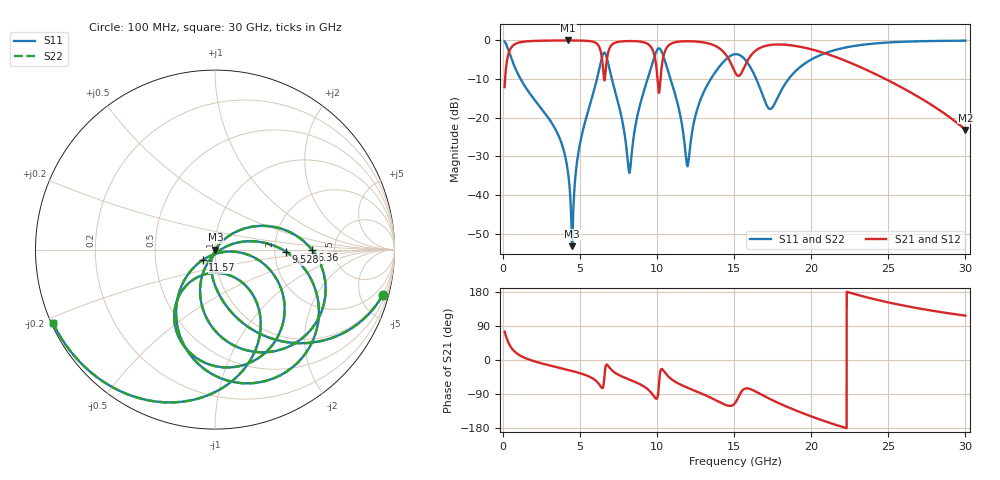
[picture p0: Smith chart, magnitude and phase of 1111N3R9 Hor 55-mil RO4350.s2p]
# GHz S MA R 50
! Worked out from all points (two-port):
!   3201 points, 100 MHz to 30 GHz, reference 50 ohm
!   highest |S21| = -0.02 dB at 4.221 GHz (marker M1); lowest = -23.2 dB at 30 GHz (marker M2)
!   |S21| within 3 dB of the highest: 388.2 MHz to 6.346 GHz (5.957 GHz wide, 177 % of centre); 16.28 GHz to 20.64 GHz (4.351 GHz wide, 23.6 % of centre)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
!   lowest |S11| = -53.3 dB at 4.482 GHz (marker M3), VSWR 1.00, Z = 50.2 - j0.11 ohm
!   |S11| at or under -10 dB: 1.14 GHz to 6.091 GHz (4.951 GHz wide, 137 % of centre); 7.061 GHz to 9.377 GHz (2.316 GHz wide, 28.2 % of centre); 10.87 GHz to 13.48 GHz (2.61 GHz wide, 21.4 % of centre)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
!   |S22| runs from -53.3 to -0.1 dB; largest |S21 - S12| = 0
!   S11 on the Smith chart (normalised r, x): 100 MHz: 0.92, -7.46; 6.36 GHz: 3.36, -0.02; 9.528 GHz: 2.31, -0.07; 11.57 GHz: 0.87, -0.10; 30 GHz: 0.00, -0.22
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0.1  0.9686 -15.0  0.2484 74.9  0.2484 74.9  0.9686 -15.0
1.081094  0.3325 -77.6  0.9424 12.3  0.9424 12.3  0.3325 -77.6
3.482438  0.0656 -107.9  0.9962 -18.9  0.9962 -18.9  0.0656 -107.9
4.220594  0.01912 -110.9  0.9975 -26.3  0.9975 -26.3  0.01912 -110.9
4.482219  0.002174 -30.4  0.9973 -29.0  0.9973 -29.0  0.002174 -30.4
5.089563  0.05712 49.7  0.9936 -36.1  0.9936 -36.1  0.05712 49.7
6.360313  0.5411 -0.2  0.6844 -71.5  0.6844 -71.5  0.5411 -0.2
6.724719  0.6008 -70.5  0.5441 -12.0  0.5441 -12.0  0.6008 -70.5
7.089125  0.3005 -105.0  0.8874 -28.0  0.8874 -28.0  0.3005 -105.0
8.191688  0.01933 -52.8  0.9798 -51.6  0.9798 -51.6  0.01933 -52.8
9.527844  0.3967 -1.8  0.8551 -82.5  0.8551 -82.5  0.3967 -1.8
10.06978  0.7833 -55.4  0.2419 -86.2  0.2419 -86.2  0.7833 -55.4
10.55566  0.5029 -113.6  0.7632 -35.8  0.7632 -35.8  0.5029 -113.6
11.57413  0.08905 -139.6  0.9698 -66.1  0.9698 -66.1  0.08905 -139.6
11.98525  0.02383 -63.4  0.9752 -73.5  0.9752 -73.5  0.02383 -63.4
12.98503  0.2067 -10.2  0.9426 -90.5  0.9426 -90.5  0.2067 -10.2
15.05  0.6623 -75.8  0.3893 -113.8  0.3893 -113.8  0.6623 -75.8
15.98438  0.4711 -118.4  0.5988 -75.9  0.5988 -75.9  0.4711 -118.4
17.32053  0.1295 -90.1  0.8714 -103.0  0.8714 -103.0  0.1295 -90.1
20.03956  0.5712 -65.2  0.7633 -149.5  0.7633 -149.5  0.5712 -65.2
25.01978  0.9395 -120.3  0.3015 151.8  0.3015 151.8  0.9395 -120.3
30  0.9913 -155.5  0.06957 117.1  0.06957 117.1  0.9913 -155.5
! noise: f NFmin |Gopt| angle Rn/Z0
0.1  0.001176  0.8558  3.688  0.001741
3.417  0.009143  0.453  23.59  0.002696
6.743  0.2362  0.9454  43.07  0.8385
10.06  0.6476  0.9707  62.42  3.68
13.39  0.1095  0.7948  80.38  0.06491
16.7  0.2474  0.8829  98.28  0.1971
20.03  0.1554  0.7912  113.5  0.04761
23.35  0.1863  0.8055  127.5  0.04084
26.67  0.2937  0.8681  142  0.05281
30  0.6718  0.9413  157.6  0.09951
